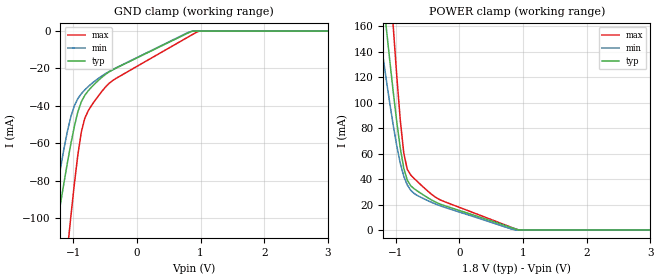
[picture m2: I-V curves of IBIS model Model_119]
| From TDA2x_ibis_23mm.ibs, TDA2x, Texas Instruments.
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| Model based on original model for DDR_SEIOPB_H
|   Sub model DDR2_ODT_60_1P8
[model]   Model_119
|[Description]  [1.8V-INPUT-X-X]
|   , ,
|[Input Load]
|[Output Drive]
|Voltage   1.8V
|Mode   INPUT
Model_type   Input
Polarity   Non-Inverting
Vinl =  0.775
Vinh =  1.025
C_comp   1p   0.5p   1.75p
[Receiver Thresholds]
Tslew_ac = 0.5n
Vth= 0.9
Vth_max= 0.945
Vth_min= 0.81
Vinh_ac= 0.2
Vinh_dc= 0.125
Vinl_ac= -0.2
Vinl_dc= -0.125
[Temperature Range]   25   125   -40
[Voltage Range]   1.8   1.71   1.89
[POWER_clamp]
-1.8V     487.3mA    361.5mA    766.2mA
-1.255V   210.7mA    155.8mA    325.3mA
-1.145V   157.9mA    117.3mA    240.2mA
-1.036V   107.6mA    81.63mA    158.4mA
-927.3mV  64.13mA    52.3mA     86.06mA
-872.7mV  48.51mA    42.14mA    60.31mA
-818.2mV  39.22mA    35.41mA    47.62mA
-763.6mV  34.73mA    31.19mA    43.2mA
-654.5mV  30.45mA    26.93mA    37.81mA
-327.3mV  20.84mA    19.47mA    24.31mA
927.3mV   112.6uA    0A         0A
3.6V      0A         0A         0A
[GND_clamp]
-1.8V     -225.3mA   -213.2mA   -377.3mA
-1.364V   -127.7mA   -109mA     -214.7mA
-1.255V   -104.1mA   -84.92mA   -175mA
-1.091V   -70.51mA   -53.64mA   -117.4mA
-1.036V   -60.27mA   -45.81mA   -99.14mA
-927.3mV  -43.31mA   -36.14mA   -66.38mA
-872.7mV  -37.87mA   -33.53mA   -54.14mA
-818.2mV  -34.42mA   -31.49mA   -46.7mA
-436.4mV  -21.86mA   -21.64mA   -27.98mA
818.2mV   -789.7uA   -517.4uA   -2.91mA
981.8mV   0A         0A         0A
3.6V      0A         0A         0A
